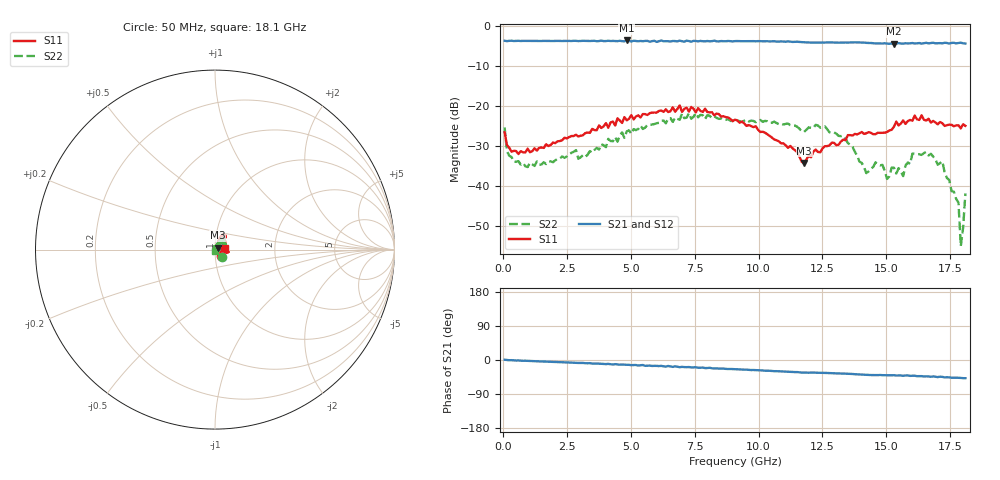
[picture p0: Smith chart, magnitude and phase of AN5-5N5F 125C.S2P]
! Network Analyzer HP8720D.06.14 Serial No. US36140669
!  5 Jul 2005  08:14:43
! Frequency  S11  S21  S12  S22
# HZ  S  DB R 50
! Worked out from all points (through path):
!   201 points, 50 MHz to 18.1 GHz, reference 50 ohm
!   highest |S21| = -3.55 dB at 4.833 GHz (marker M1); lowest = -4.4 dB at 15.3 GHz (marker M2)
!   group delay of S21, straight-line fit = 7.45 ps
!   lowest |S11| = -34.3 dB at 11.78 GHz (marker M3), VSWR 1.04, Z = 51.6 + j1.19 ohm
!   |S11| at or under -10 dB: start of sweep to end of sweep
!   |S22| runs from -55.2 to -21.8 dB; largest |S21 - S12| = 0.019
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5e7  -26.61 -48.1  -3.62 0.7  -3.66 0.8  -25.34 -47.7
1.4025e8  -29.77 -32.4  -3.71 0.0  -3.70 -0.1  -31.32 -38.3
2.305e8  -30.47 -22.0  -3.65 -0.6  -3.63 -0.5  -32.46 -32.0
8.6225e8  -31.65 -6.5  -3.66 -2.0  -3.69 -2.0  -35.13 -3.6
3.1185e9  -27.33 21.5  -3.64 -7.7  -3.67 -7.9  -32.34 42.1
4.83325e9  -23.60 46.1  -3.55 -12.7  -3.64 -12.8  -26.37 50.5
6.09675e9  -21.24 50.1  -3.73 -16.0  -3.65 -16.0  -24.22 55.8
7.27e9  -21.39 58.2  -3.71 -18.6  -3.78 -19.7  -21.79 54.4
9.075e9  -23.42 66.4  -3.71 -24.3  -3.69 -24.4  -23.60 38.2
1.17825e10  -34.31 36.7  -4.01 -33.0  -4.00 -33.3  -26.49 50.5
1.21435e10  -31.45 37.4  -4.10 -33.0  -4.05 -33.3  -25.52 58.9
1.331675e10  -28.45 4.0  -4.05 -35.8  -4.06 -36.0  -27.46 67.0
1.421925e10  -26.84 -29.8  -4.15 -38.9  -4.15 -39.1  -36.84 104.6
1.458025e10  -27.06 -27.5  -4.30 -40.0  -4.24 -40.2  -34.15 116.0
1.512175e10  -26.15 -13.3  -4.37 -40.6  -4.29 -40.5  -37.64 107.7
1.530225e10  -25.19 -15.4  -4.38 -40.1  -4.30 -41.2  -35.51 109.6
1.566325e10  -23.60 -11.6  -4.35 -41.7  -4.27 -40.9  -37.60 66.8
1.602425e10  -23.70 -11.4  -4.19 -41.5  -4.33 -42.6  -31.95 35.1
1.71975e10  -24.34 -2.6  -4.27 -44.5  -4.20 -43.8  -33.89 -14.9
1.782925e10  -24.84 8.6  -4.18 -47.0  -4.20 -46.7  -44.26 -56.5
1.79195e10  -25.63 6.8  -4.11 -47.3  -4.02 -47.0  -55.17 -47.2
1.81e10  -24.99 8.3  -4.33 -48.0  -4.34 -48.7  -41.90 -103.4
